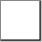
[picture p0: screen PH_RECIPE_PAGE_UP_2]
VISUALIZATION PH_RECIPE_PAGE_UP_2  // 42x42
VAR_IN_OUT
	RECIPE_CTRL_V2 : None;
END_VAR
    Rectangle (0,0 40x40)
        tap RECIPE_CTRL_V2.sCmd.bPageUp
    Polygon (20,20), colour toggle: (RECIPE_CTRL_V2.sCmd.bPageUp) <> 0
        tap RECIPE_CTRL_V2.sCmd.bPageUp
    Polygon (20,10), colour toggle: (RECIPE_CTRL_V2.sCmd.bPageUp) <> 0
        tap RECIPE_CTRL_V2.sCmd.bPageUp
END_VISUALIZATION
